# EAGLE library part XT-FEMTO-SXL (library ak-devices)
AK-NORD XT-FEMTO-SXL
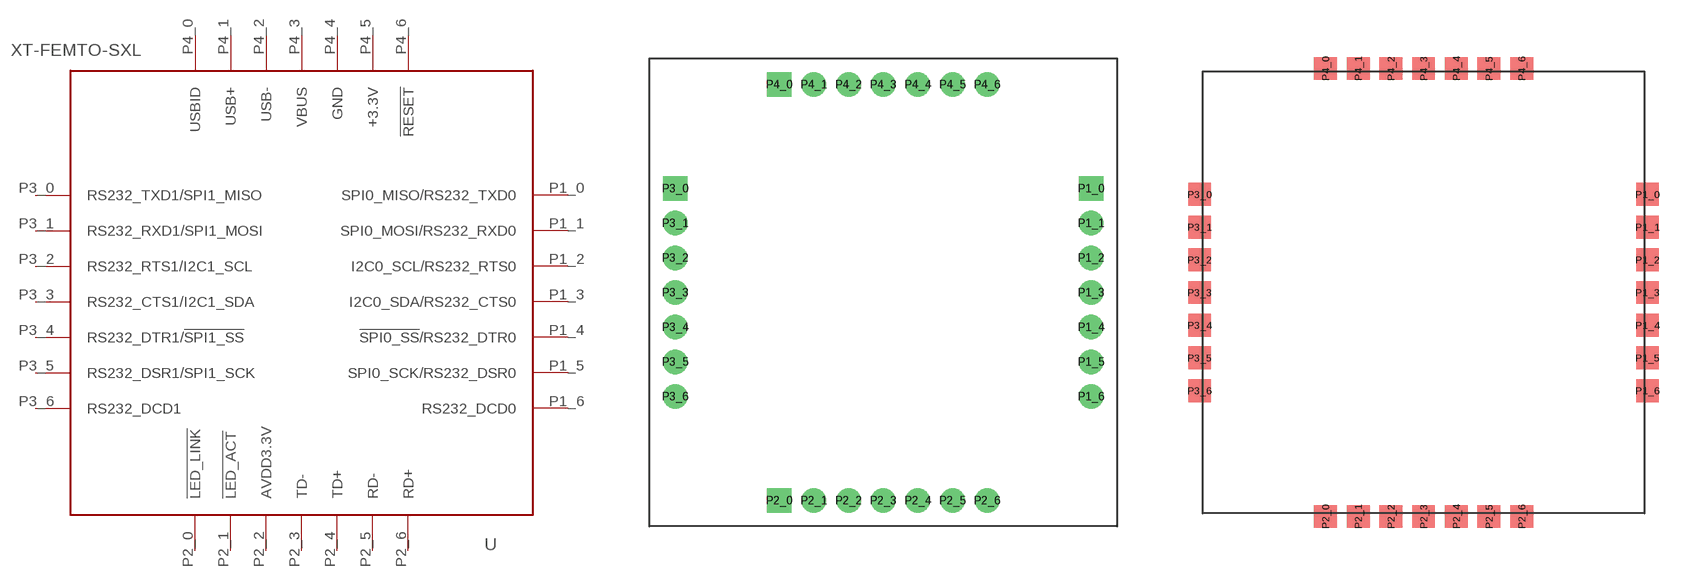
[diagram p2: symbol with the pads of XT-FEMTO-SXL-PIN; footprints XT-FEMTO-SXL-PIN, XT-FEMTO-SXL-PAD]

Designator prefix -

## XT-FEMTO-SXL1  [XT-FEMTO-SXL-PIN]
P1_0  SPI0_MISO/RS232_TXD0
P1_1  SPI0_MOSI/RS232_RXD0
P1_2  I2C0_SCL/RS232_RTS0
P1_3  I2C0_SDA/RS232_CTS0
P1_4  !SPI0_SS!/RS232_DTR0
P1_5  SPI0_SCK/RS232_DSR0
P1_6  RS232_DCD0
P2_0  !LED_LINK  out
P2_1  !LED_ACT  out
P2_2  AVDD3.3V  pas
P2_3  TD-  pas
P2_4  TD+  pas
P2_5  RD-  pas
P2_6  RD+  pas
P3_0  RS232_TXD1/SPI1_MISO
P3_1  RS232_RXD1/SPI1_MOSI
P3_2  RS232_RTS1/I2C1_SCL
P3_3  RS232_CTS1/I2C1_SDA
P3_4  RS232_DTR1/!SPI1_SS!
P3_5  RS232_DSR1/SPI1_SCK
P3_6  RS232_DCD1
P4_0  USBID  pas
P4_1  USB+  pas
P4_2  USB-  pas
P4_3  VBUS  pas
P4_4  GND  pwr
P4_5  +3.3V  pwr
P4_6  !RESET  pas

## XT-FEMTO-SXL2  [XT-FEMTO-SXL-PAD]
Pads as for XT-FEMTO-SXL-PIN

## Footprint XT-FEMTO-SXL-PIN (pad centres in mm)
AK-NORD XT-FEMTO-SXL
drill 0.813 pad 1.422 square: P1_0 12,6; P2_0 -6,-12; P3_0 -12,6; P4_0 -6,12
drill 0.813 pad 1.422: P1_1 12,4; P1_2 12,2; P1_3 12,0; P1_4 12,-2; P1_5 12,-4; P1_6 12,-6; P2_1 -4,-12; P2_2 -2,-12; P2_3 0,-12; P2_4 2,-12; P2_5 4,-12; P2_6 6,-12; P3_1 -12,4; P3_2 -12,2; P3_3 -12,0; P3_4 -12,-2; P3_5 -12,-4; P3_6 -12,-6; P4_1 -4,12; P4_2 -2,12; P4_3 0,12; P4_4 2,12; P4_5 4,12; P4_6 6,12

## Footprint XT-FEMTO-SXL-PAD (pad centres in mm)
smd 1.4 x 1.4: P1_0 13.7,6; P1_1 13.7,4; P1_2 13.7,2; P1_3 13.7,0; P1_4 13.7,-2; P1_5 13.7,-4; P1_6 13.7,-6; P2_0 -6,-13.7; P2_1 -4,-13.7; P2_2 -2,-13.7; P2_3 0,-13.7; P2_4 2,-13.7; P2_5 4,-13.7; P2_6 6,-13.7; P3_0 -13.7,6; P3_1 -13.7,4; P3_2 -13.7,2; P3_3 -13.7,0; P3_4 -13.7,-2; P3_5 -13.7,-4; P3_6 -13.7,-6; P4_0 -6,13.7; P4_1 -4,13.7; P4_2 -2,13.7; P4_3 0,13.7; P4_4 2,13.7; P4_5 4,13.7; P4_6 6,13.7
